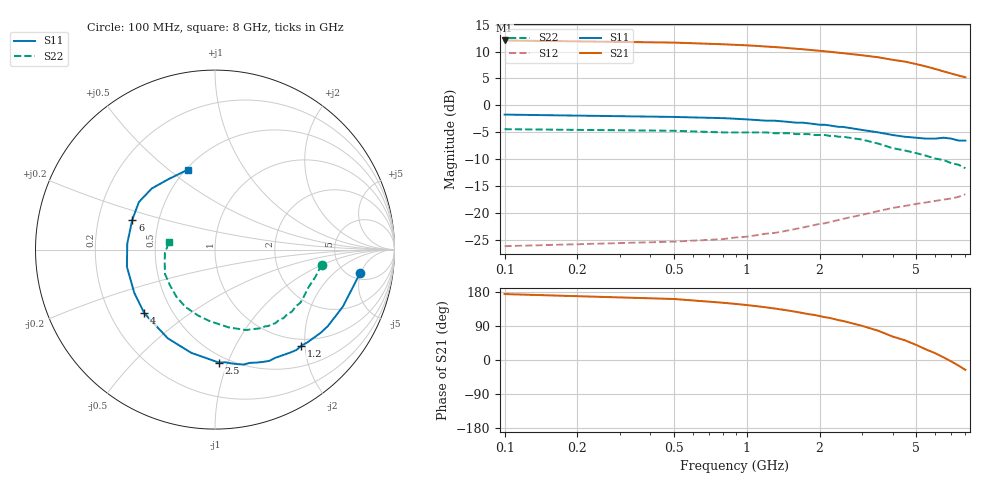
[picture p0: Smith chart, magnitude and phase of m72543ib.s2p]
!  MGA-72543 S PARAMETERS
!  Vd=3V  Id=5 mA Vc=0.7V  LAST UPDATED 01-27-99
# ghz s ma r 50
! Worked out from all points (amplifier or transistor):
!   31 points, 100 MHz to 8 GHz, reference 50 ohm
!   highest |S21| = 12.1 dB at 100 MHz (marker M1)
!   |S21| within 3 dB of that: start of sweep to 3.319 GHz
!   unconditionally stable (mu >= 1): start of sweep to 2.471 GHz; 2.643 GHz to end of sweep
!   at 1.1 GHz: K = 1.07, MAG = 16.0 dB, |S12| = -24.2 dB
!   at 2.1 GHz: K = 1.00, MAG = 15.6 dB, |S12| = -21.9 dB
!   at 8 GHz: K = 1.35, MAG = 7.3 dB, |S12| = -16.5 dB
!   lowest NFmin = 1.43 dB at 1 GHz
!   S11 on the Smith chart (normalised r, x): 100 MHz: 6.23, -4.88; 1.2 GHz: 0.87, -1.93; 2.5 GHz: 0.45, -0.93; 4 GHz: 0.35, -0.34; 6 GHz: 0.35, +0.16; 8 GHz: 0.51, +0.58
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0.1  0.82 -9.0  4.012 174.0  0.049 19.0  0.6 -8.0
0.5  0.78 -24.0  3.833 161.0  0.054 13.0  0.58 -15.0
0.8  0.76 -34.0  3.696 151.0  0.057 15.0  0.56 -23.0
0.9  0.75 -38.0  3.652 148.0  0.059 16.0  0.56 -26.0
1.2  0.72 -48.0  3.523 139.0  0.064 18.0  0.56 -32.0
1.4  0.71 -54.0  3.445 133.0  0.067 19.0  0.55 -37.0
1.8  0.68 -67.0  3.286 121.0  0.075 18.0  0.54 -45.0
1.9  0.67 -70.0  3.248 119.0  0.077 18.0  0.53 -47.0
2.1  0.66 -76.0  3.179 113.0  0.08 17.0  0.53 -51.0
2.2  0.65 -79.0  3.15 111.0  0.082 16.0  0.52 -53.0
2.4  0.63 -85.0  3.083 105.0  0.086 15.0  0.51 -57.0
2.5  0.63 -88.0  3.056 103.0  0.088 15.0  0.51 -59.0
3  0.59 -103.0  2.92 90.0  0.096 11.0  0.48 -69.0
3.5  0.56 -118.0  2.796 77.0  0.104 7.0  0.44 -80.0
4  0.53 -138.0  2.652 62.0  0.111 1.0  0.4 -94.0
4.5  0.51 -152.0  2.552 52.0  0.116 -3.0  0.38 -104.0
5  0.5 -169.0  2.421 40.0  0.121 -9.0  0.36 -117.0
5.5  0.49 176.0  2.3 28.0  0.125 -13.0  0.34 -129.0
6  0.49 160.0  2.18 18.0  0.129 -17.0  0.32 -142.0
6.5  0.5 148.0  2.07 7.0  0.133 -23.0  0.31 -154.0
7  0.49 136.0  1.975 -4.0  0.136 -28.0  0.29 -165.0
8  0.47 109.0  1.825 -26.0  0.149 -37.0  0.26 171.0
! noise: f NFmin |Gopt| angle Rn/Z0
0.8  1.58  0.59  31  0.34
1  1.43  0.46  37  0.32
1.8  1.67  0.31  55  0.3
2  1.68  0.29  60  0.28
2.2  1.72  0.29  66  0.27
2.4  1.74  0.28  71  0.26
3  1.78  0.25  87  0.24
4  1.83  0.22  121  0.18
5  1.87  0.22  164  0.15
6  1.94  0.26  -150  0.15
